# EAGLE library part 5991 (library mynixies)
B-5991 or HP 1970-0009 Nixie Tube
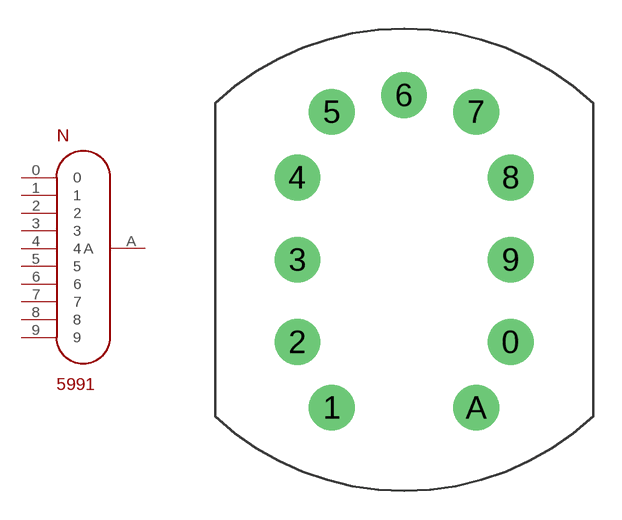
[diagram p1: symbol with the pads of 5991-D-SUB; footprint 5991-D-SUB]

Designator prefix N

## 59915991-D-SUB  [5991-D-SUB]
0  0  pas
1  1  pas
2  2  pas
3  3  pas
4  4  pas
5  5  pas
6  6  pas
7  7  pas
8  8  pas
9  9  pas
A  A  pas

## Footprint 5991-D-SUB (pad centres in mm)
drill 1.6: 0 5.588,-4.318; 1 -3.786,-7.762; 2 -5.588,-4.318; 3 -5.588,0; 4 -5.588,4.318; 5 -3.786,7.762; 6 0,8.636; 7 3.786,7.762; 8 5.588,4.318; 9 5.588,0; A 3.786,-7.762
